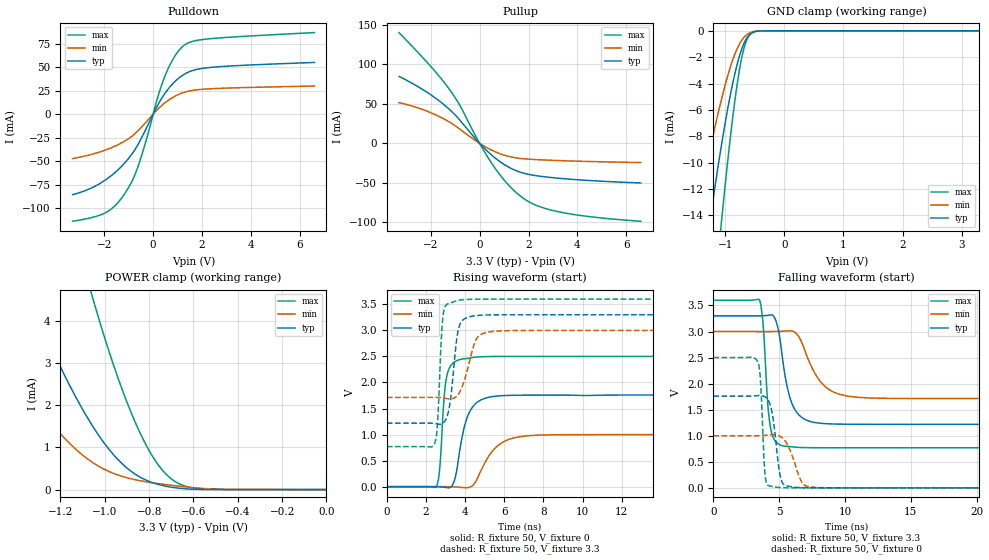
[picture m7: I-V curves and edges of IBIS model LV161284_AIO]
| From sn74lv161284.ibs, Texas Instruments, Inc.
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[Model]   LV161284_AIO
Model_type  I/O
Vinl=0.8
Vinh=2.0
Enable   Active-High
Vref =   0
Rref =   500
Cref =   50p
Vmeas =   1.4
| variable   typ   min   max
C_comp   3.62pF   3.13pF   3.85pF
| C_pullup   5.05pF   3.25pF   6.30pF
| C_pulldown   4.97pF   3.68pF   6.49pF
| C_tri-state   3.62pF   3.13pF   3.85pF
[Temperature Range]   40   100   -40
| Ambient temperature   25   85   -40
[Voltage range]   3.3   3   3.6
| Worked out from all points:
|   slope of the pulldown table from 0 to 0.495 V, typ, clamps not added: 21.9 ohm
|   slope of the pullup table from 0 to 0.495 V, typ, clamps not added: 32.9 ohm
|   GND clamp passes 1 mA (typ) near -0.69 V on its own axis
|   POWER clamp passes 1 mA (typ) near -0.99 V on its own axis
|   rising waveform, R_fixture 50, V_fixture 0: 20-80 % time 602ps typ, 1.04ns min, 274ps max; typ from 0 V to 1.76 V
|   falling waveform, R_fixture 50, V_fixture 3.3: 20-80 % time 901ps typ, 1.59ns min, 430ps max; typ from 3.3 V to 1.22 V
|   rising waveform, R_fixture 50, V_fixture 3.3: 20-80 % time 353ps typ, 569ps min, 206ps max; typ from 1.22 V to 3.3 V
|   falling waveform, R_fixture 50, V_fixture 0: 20-80 % time 507ps typ, 856ps min, 265ps max; typ from 1.76 V to 0 V
[GND Clamp]
| LV161284_AIO
|   Voltage   I(typ)   I(min)   I(max)
-3.3V     -104.8mA   -68.09mA   -142.4mA
-1.53V    -23.95mA   -15.19mA   -37.99mA
-1.49V    -22.48mA   -14.23mA   -35.83mA
-1.255V   -14.4mA    -8.956mA   -23.63mA
-1.08V    -9.121mA   -5.495mA   -15.22mA
-1.05V    -8.291mA   -4.953mA   -13.86mA
-920mV    -5.009mA   -2.843mA   -8.35mA
-785mV    -2.312mA   -1.224mA   -3.661mA
-695mV    -1.078mA   -563.6uA   -1.526mA
-595mV    -316.5uA   -186.1uA   -360.8uA
-380mV    -6.736uA   -5.064uA   -3.387uA
3.3V      16.78nA    35.15nA    81.44nA
[POWER Clamp]
| LV161284_AIO
|   Voltage   I(typ)   I(min)   I(max)
-3.3V     48.97mA    30.44mA    83.98mA
-1.615V   8.681mA    4.667mA    18.31mA
-1.365V   4.931mA    2.45mA     11.4mA
-1.325V   4.407mA    2.149mA    10.4mA
-1.085V   1.767mA    757.2uA    5.122mA
-1.05V    1.467mA    627.3uA    4.469mA
-945mV    737.5uA    354.6uA    2.719mA
-845mV    308.6uA    216.1uA    1.391mA
-780mV    156.5uA    158.5uA    749.6uA
-700mV    57.65uA    102.8uA    254.9uA
-550mV    2.316uA    24.67uA    11.63uA
-48.03fV  16.78nA    2.46nA     127.1nA
[Pulldown]
| LV161284_AIO
|   Voltage   I(typ)   I(min)   I(max)
-3.3V     -85.73mA   -47.31mA   -114.1mA
-1.91V    -69.26mA   -37.81mA   -104.3mA
-1.505V   -60.86mA   -33.35mA   -95.98mA
-1.1V     -50.09mA   -27.62mA   -82.15mA
-810mV    -40.28mA   -22.25mA   -68.26mA
-580mV    -30.37mA   -16.66mA   -52.75mA
185mV     9.498mA    5.169mA    17.88mA
470mV     21.64mA    11.85mA    39.72mA
855mV     33.85mA    18.6mA     60.46mA
1.25V     42.13mA    23.1mA     73.01mA
2.385V    49.87mA    27.09mA    80.47mA
6.6V      55.06mA    29.96mA    86.89mA
[Pullup]
| LV161284_AIO
|   Voltage   I(typ)   I(min)   I(max)
-3.3V     84.92mA    51.7mA     140.5mA
-2.18V    65.3mA     41.13mA    103.7mA
-1.305V   44.91mA    28.3mA     71.29mA
-825mV    29.99mA    18.36mA    48.92mA
-30mV     1.024mA    612.1uA    1.679mA
500mV     -15.17mA   -8.775mA   -25.56mA
1.085V    -28.33mA   -15.66mA   -49.51mA
1.665V    -36.58mA   -19.12mA   -66.77mA
2.315V    -41mA      -20.58mA   -78.56mA
3.23V     -44.23mA   -21.82mA   -86.73mA
4.615V    -47.33mA   -23.09mA   -93.33mA
6.6V      -50.23mA   -24.33mA   -98.82mA
[Ramp]
| LV161284_AIO
| variable   typ   min   max
dV/dt_r   1.07/6.12E-10   0.61/1.04E-09   1.51/2.89E-10
dV/dt_f   1.26/9.06E-10   0.78/1.59E-09   1.71/4.38E-10
R_load = 50
[Rising Waveform]
| LV161284_AIO
R_fixture =   50
C_fixture =   0
L_fixture =   0
V_fixture =   0
V_fixture_min = 0
V_fixture_max = 0
|   Time   V(typ)   V(min)   V(max)
0s        10.57nV    4.37nV     48.01nV
2.525ns   1.443mV    108.4uV    1.723mV
2.685ns   -1.1mV     609.3uV    304.3mV
2.94ns    -11.19mV   1.003mV    1.786V
3.11ns    -20.72mV   547uV      2.2V
4.075ns   1.3V       -20.15mV   2.459V
4.56ns    1.603V     111.7mV    2.487V
5.77ns    1.744V     817.5mV    2.5V
7.82ns    1.758V     990.3mV    2.501V
70ns      1.76V      999.8mV    2.501V
[Falling Waveform]
| LV161284_AIO
R_fixture =   50
C_fixture =   0
L_fixture =   0
V_fixture =   3.3
V_fixture_min = 3
V_fixture_max = 3.6
|   Time   V(typ)   V(min)   V(max)
0s        3.3V       3V         3.6V
3.505ns   3.3V       3V         3.599V
3.765ns   3.303V     3V         3.158V
4.315ns   3.317V     3V         1.187V
4.865ns   3.103V     3.002V     854.5mV
5.39ns    2.229V     3.007V     800.9mV
6.72ns    1.35V      2.787V     774.2mV
8.39ns    1.234V     1.967V     769.8mV
11ns      1.22V      1.737V     769.5mV
70ns      1.219V     1.714V     769.4mV
[Rising Waveform]
| LV161284_AIO
R_fixture =   50
C_fixture =   0
L_fixture =   0
V_fixture =   3.3
V_fixture_min = 3
V_fixture_max = 3.6
|   Time   V(typ)   V(min)   V(max)
0s        1.219V     1.714V     769.4mV
2.405ns   1.216V     1.715V     802.5mV
2.575ns   1.204V     1.715V     1.152V
2.9ns     1.231V     1.702V     3.364V
3.18ns    1.508V     1.685V     3.52V
3.58ns    2.867V     1.742V     3.571V
3.825ns   3.177V     1.899V     3.587V
4.605ns   3.286V     2.856V     3.598V
5.815ns   3.299V     2.991V     3.6V
70ns      3.3V       3V         3.6V
[Falling Waveform]
| LV161284_AIO
R_fixture =   50
C_fixture =   0
L_fixture =   0
V_fixture =   0
V_fixture_min = 0
V_fixture_max = 0
|   Time   V(typ)   V(min)   V(max)
0s        1.76V      999.8mV    2.501V
3.345ns   1.77V      999.8mV    2.43V
3.56ns    1.773V     1.002V     2.11V
3.975ns   1.735V     1.01V      153.7mV
4.41ns    1.503V     1.018V     29.68mV
4.77ns    827.8mV    1.014V     13.27mV
5.305ns   72.01mV    943.3mV    3.542mV
6.735ns   4.333mV    102.1mV    221.2uV
7.785ns   826.7uV    8.859mV    38.3uV
70ns      162.3nV    474.3nV    111.1nV
